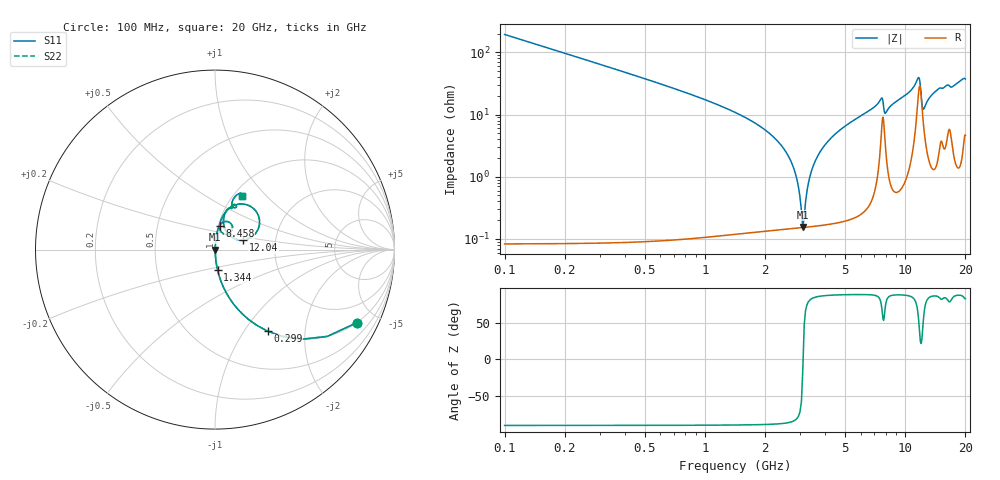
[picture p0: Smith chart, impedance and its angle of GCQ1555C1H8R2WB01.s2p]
!Murata Part Number: GCQ1555C1H8R2WB01
!These Parameters are Measured in Series Mode Connection
!Data Generated on Mar 13, 2026
!  o--ll--o
!Port1  Port2
!  o------o
!Operation Temp=25[degC], DC Bias Voltage=0[V]
!Freq. Start=100[MHz] Stop=20[GHz] 401[Steps]
# Hz S RI R 50
!Freq.(Hz) S11(Real) S11(Imag) S21(Real) S21(Imag) S12(Real) S12(Imag) S22(Real) S22(Imag)
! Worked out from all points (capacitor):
!   401 points, 100 MHz to 20 GHz, reference 50 ohm
!   read as one part in series: C = 8.2 pF near 199.5 MHz
!   lowest |Z| = 156 mohm at 3.085 GHz (marker M1)
!   series resonance near 3.094 GHz, so ESL is about 320 pH
!   S11 on the Smith chart (normalised r, x): 100 MHz: 1.00, -3.88; 299 MHz: 1.00, -1.29; 1.344 GHz: 1.00, -0.23; 8.458 GHz: 1.01, +0.27; 12.04 GHz: 1.37, +0.15; 20 GHz: 1.09, +0.74
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1e8  0.7898 -0.4073  0.2102 0.4073  0.2102 0.4073  0.7898 -0.4073
2.99e8  0.2928 -0.4544  0.7072 0.4544  0.7072 0.4544  0.2928 -0.4544
5.975e8  0.0897 -0.2843  0.9103 0.2843  0.9103 0.2843  0.0897 -0.2843
1.34375e9  0.0147 -0.1153  0.9853 0.1153  0.9853 0.1153  0.0147 -0.1153
2.5875e9  0.00195 -0.0226  0.9981 0.0226  0.9981 0.0226  0.00195 -0.0226
2.83625e9  0.0016 -0.0109  0.9984 0.0109  0.9984 0.0109  0.0016 -0.0109
3.085e9  0.00152 -0.000352  0.9985 0.000352  0.9985 0.000352  0.00152 -0.000352
3.1845e9  0.00155 0.00365  0.9984 -0.00365  0.9984 -0.00365  0.00155 0.00365
3.43325e9  0.00175 0.0132  0.9982 -0.0132  0.9982 -0.0132  0.00175 0.0132
3.83125e9  0.0024 0.0273  0.9976 -0.0273  0.9976 -0.0273  0.0024 0.0273
4.42825e9  0.00396 0.0468  0.996 -0.0468  0.996 -0.0468  0.00396 0.0468
6.7665e9  0.0183 0.1185  0.9817 -0.1185  0.9817 -0.1185  0.0183 0.1185
7.61225e9  0.0736 0.1552  0.9264 -0.1552  0.9264 -0.1552  0.0736 0.1552
7.9605e9  0.0411 0.0919  0.9589 -0.0919  0.9589 -0.0919  0.0411 0.0919
8.458e9  0.0254 0.1324  0.9746 -0.1324  0.9746 -0.1324  0.0254 0.1324
1.005e10  0.0481 0.1939  0.9519 -0.1939  0.9519 -0.1939  0.0481 0.1939
1.159225e10  0.2144 0.2292  0.7856 -0.2292  0.7856 -0.2292  0.2144 0.2292
1.204e10  0.1585 0.0532  0.8415 -0.0532  0.8415 -0.0532  0.1585 0.0532
1.23385e10  0.0744 0.0851  0.9256 -0.0851  0.9256 -0.0851  0.0744 0.0851
1.338325e10  0.0499 0.1821  0.9501 -0.1821  0.9501 -0.1821  0.0499 0.1821
1.67165e10  0.1149 0.2337  0.8851 -0.2337  0.8851 -0.2337  0.1149 0.2337
2e10  0.1507 0.3005  0.8493 -0.3005  0.8493 -0.3005  0.1507 0.3005
